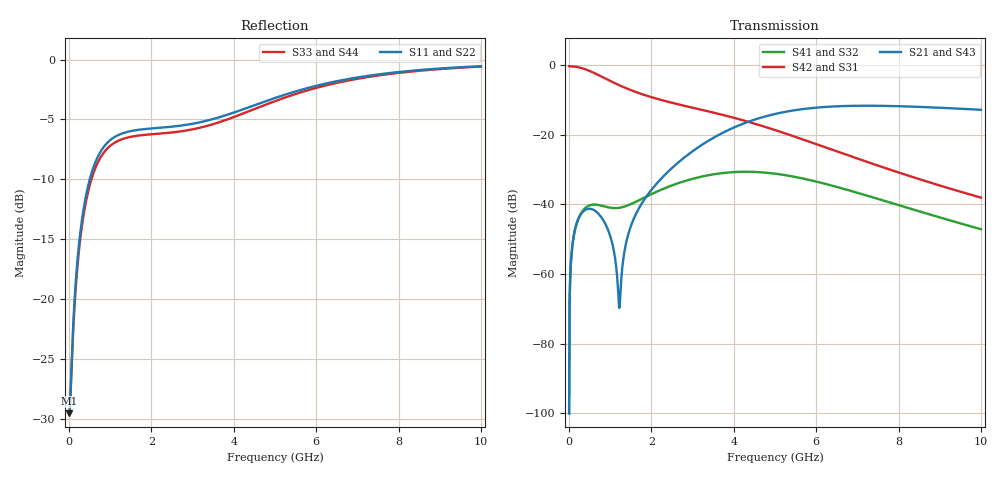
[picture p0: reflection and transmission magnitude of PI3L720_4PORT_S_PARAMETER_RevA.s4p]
! NPort=4 DATA=800 NOISE=0 GROUPDELAY=0 COMPLEX_DATAFORMAT=POLAR
! NumOfBlock=1 NumOfParam=0
! .MODEL Smodel S TSTONEFILE=PI3L720_4PORT_S_PARAMETER_RevA.s4p TYPE=S
!  -- The above .MODEL line can be used for the S element in the netlist.
!Port definition:
!Port1 = input+
!Port2 = input¨C
!Port3 = output+
!Port4 = output-
# Hz S MA R  50
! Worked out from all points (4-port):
!   800 points, 300 kHz to 10 GHz, reference 50 ohm
!   strongest paths, dB at 300 kHz, 2.503 GHz, 5.006 GHz, 7.509 GHz, 10 GHz:
!     S21: -100.0, -29.5, -14.0, -11.7, -12.8
!     S43: -100.0, -29.5, -14.2, -11.8, -12.9
!     S42: -0.3, -10.8, -18.7, -28.9, -38.1
!     S31: -0.3, -10.8, -18.7, -28.9, -38.1
!     S41: -100.0, -34.5, -31.2, -38.5, -47.1
!     S32: -100.0, -34.5, -31.2, -38.5, -47.1
!   lowest |S11| = -29.5 dB at 300 kHz (marker M1), VSWR 1.07, Z = 53.5 - j0.0309 ohm
!   |S11| at or under -10 dB: start of sweep to 501.4 MHz
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300000  0.03335 -0.5  9.964e-06 89.9  0.9666 -0.0  9.945e-06 89.9
        9.964e-06 89.9  0.03335 -0.5  9.945e-06 89.9  0.9666 -0.0
        0.9666 -0.0  9.945e-06 89.9  0.03335 -0.5  9.964e-06 89.9
        9.945e-06 89.9  0.9666 -0.0  9.964e-06 89.9  0.03335 -0.5
1.12937e8  0.08626 -80.1  0.003517 70.8  0.9557 -10.4  0.003528 70.6
           0.003517 70.8  0.08626 -80.1  0.003528 70.6  0.9557 -10.4
           0.9558 -10.4  0.003528 70.6  0.08205 -79.0  0.003517 71.1
           0.003528 70.6  0.9558 -10.4  0.003517 71.1  0.08205 -79.0
3.75758e8  0.2512 -119.1  0.008208 37.3  0.8795 -33.4  0.008698 37.4
           0.008208 37.3  0.2512 -119.1  0.008698 37.4  0.8795 -33.4
           0.8795 -33.4  0.008699 37.4  0.2374 -118.7  0.008215 38.2
           0.008699 37.4  0.8795 -33.4  0.008215 38.2  0.2374 -118.7
1.21428e9  0.4858 174.5  0.0003249 -85.6  0.5158 -83.9  0.008918 8.7
           0.0003249 -85.6  0.4858 174.5  0.008918 8.7  0.5158 -83.9
           0.516 -83.8  0.00892 8.7  0.4599 174.3  0.0001219 81.9
           0.00892 8.7  0.516 -83.8  0.0001219 81.9  0.4599 174.3
1.67735e9  0.5089 149.6  0.008376 165.7  0.4 -100.8  0.0113 12.0
           0.008376 165.7  0.5089 149.6  0.0113 12.0  0.4 -100.8
           0.4002 -100.8  0.01131 12.0  0.4815 149.2  0.008621 160.7
           0.01131 12.0  0.4002 -100.8  0.008621 160.7  0.4815 149.2
3.29182e9  0.553 72.8  0.07591 139.3  0.2225 -151.4  0.02554 -37.5
           0.07591 139.3  0.553 72.8  0.02554 -37.5  0.2225 -151.4
           0.2228 -151.3  0.02558 -37.5  0.5253 71.5  0.07486 136.8
           0.02558 -37.5  0.2228 -151.3  0.07486 136.8  0.5253 71.5
1e10  0.9386 -96.2  0.2285 -4.0  0.01247 70.4  0.004387 110.7
      0.2285 -4.0  0.9386 -96.2  0.004387 110.7  0.01247 70.4
      0.0125 70.4  0.004397 110.7  0.9351 -96.3  0.2276 -3.8
      0.004397 110.7  0.0125 70.4  0.2276 -3.8  0.9351 -96.3
